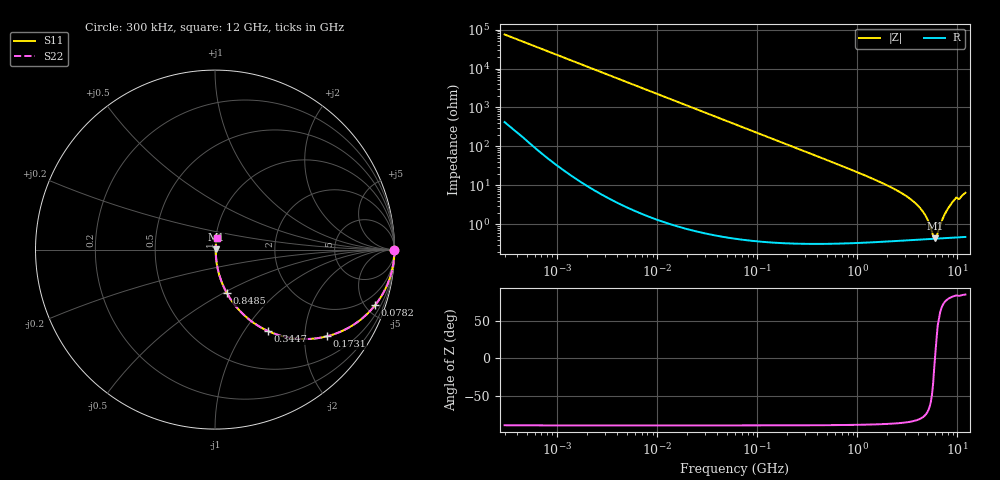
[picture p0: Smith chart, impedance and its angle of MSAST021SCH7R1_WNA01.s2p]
! MSAST021SCH7R1_WNA01  S-PARAMETER MODEL  ( General Type )
! Model Generated by TAIYO YUDEN Corporation (http://www.ty-top.com)
! Version 2.0
! TAIYO YUDEN Control No. 181101
! Copyright(c) 2015 TAIYO YUDEN CO.,LTD. All Rights Reserved.
! Product Description (link to TY-COMPAS)
! https://ds.yuden.co.jp/TYCOMPAS/or/detail?pn=MSAST021SCH7R1CWNA01&u=M
! Products Name : Multilayer Ceramic Capacitors
! Characteristics :
!  Capacitance : 7.1 pF , Rated Voltage : 25V , TCC : CH / C0H
!  Case Size : 0.25 x 0.125 / 0.0098 x 0.0049 [mm/inch] , Thickness : 0.125 / 0.0049 [mm/inch]
!  (Conditions: Temperature = 25 degC , DC Bias Current/Voltage = 0A / 0V)
! External Node Assignments :
!  1  o---| |---o  2
! GND o---------o GND
! Frequency Range : 0.3MHz  -  12000MHz  [ 401 STEP ]
# MHz S RI R 50
! Freq[MHz].  S11 Real  S11 Imag  S21 Real  S21 Imag  S12 Real  S12 Imag  S22 Real  S22 Imag
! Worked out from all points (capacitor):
!   401 points, 300 kHz to 12 GHz, reference 50 ohm
!   read as one part in series: C = 7.1 pF near 316.3 kHz
!   lowest |Z| = 437 mohm at 6.026 GHz (marker M1)
!   series resonance near 5.957 GHz, so ESL is about 100 pH
!   S11 on the Smith chart (normalised r, x): 300 kHz: open; 78.2 MHz: 1.01, -5.73; 173.1 MHz: 1.01, -2.59; 344.7 MHz: 1.01, -1.30; 848.5 MHz: 1.01, -0.52; 12 GHz: 1.01, +0.13
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0.3  1 -0.00134  9.33e-06 0.00134  9.33e-06 0.00134  1 -0.00134
1.769972  0.9999 -0.0079  6.97e-05 0.0079  6.97e-05 0.0079  0.9999 -0.0079
10.44266  0.9978 -0.0465  0.00219 0.0465  0.00219 0.0465  0.9978 -0.0465
27.10171  0.9855 -0.1191  0.0145 0.1191  0.0145 0.1191  0.9855 -0.1191
60  0.9329 -0.2496  0.0671 0.2496  0.0671 0.2496  0.9329 -0.2496
78.19928  0.8911 -0.3108  0.1089 0.3108  0.1089 0.3108  0.8911 -0.3108
173.124  0.6257 -0.4827  0.3743 0.4827  0.3743 0.4827  0.6257 -0.4827
344.7396  0.2967 -0.4544  0.7033 0.4544  0.7033 0.4544  0.2967 -0.4544
353.9943  0.2857 -0.4493  0.7143 0.4493  0.7143 0.4493  0.2857 -0.4493
848.5281  0.0654 -0.2411  0.9346 0.2411  0.9346 0.2411  0.0654 -0.2411
2088.533  0.0123 -0.0925  0.9877 0.0925  0.9877 0.0925  0.0123 -0.0925
3107.553  0.00658 -0.0518  0.9934 0.0518  0.9934 0.0518  0.00658 -0.0518
4050.141  0.0049 -0.0293  0.9951 0.0293  0.9951 0.0293  0.0049 -0.0293
4747.894  0.00443 -0.0169  0.9956 0.0169  0.9956 0.0169  0.00443 -0.0169
5140.631  0.00431 -0.0108  0.9957 0.0108  0.9957 0.0108  0.00431 -0.0108
5715.274  0.00427 -0.00282  0.9957 0.00282  0.9957 0.00282  0.00427 -0.00282
6026.253  0.0043 0.000661  0.9957 -0.000661  0.9957 -0.000661  0.0043 0.000661
6354.153  0.00435 0.00425  0.9957 -0.00425  0.9957 -0.00425  0.00435 0.00425
7448.838  0.00474 0.0174  0.9953 -0.0174  0.9953 -0.0174  0.00474 0.0174
8503.825  0.00547 0.0308  0.9945 -0.0308  0.9945 -0.0308  0.00547 0.0308
9454.42  0.00654 0.0441  0.9935 -0.0441  0.9935 -0.0441  0.00654 0.0441
12000  0.00884 0.0638  0.9912 -0.0638  0.9912 -0.0638  0.00884 0.0638
